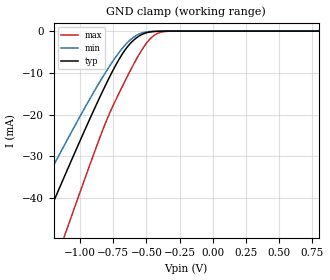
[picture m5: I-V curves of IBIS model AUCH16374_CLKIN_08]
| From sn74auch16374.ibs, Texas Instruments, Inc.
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[Model]   AUCH16374_CLKIN_08
Model_type  Input
Vinl=0
Vinh=0.8
| variable   typ   min   max
C_comp   2.55pF   2.23pF   2.86pF
[Temperature Range]   40   100   -40
| Ambient temperature   25   85   -40
[Voltage range]   0.8   0.8   0.8
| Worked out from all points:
|   GND clamp passes 1 mA (typ) near -0.55 V on its own axis
[GND Clamp]
| AUCH16374_CLKIN_08
|   Voltage   I(typ)   I(min)   I(max)
-3.6V     -222.3mA   -186.1mA   -267.5mA
-1.455V   -59.66mA   -47.61mA   -78.99mA
-1.32V    -49.56mA   -39.31mA   -66.95mA
-1.275V   -46.22mA   -36.57mA   -62.93mA
-1.115V   -34.43mA   -26.99mA   -48.63mA
-1.08V    -31.88mA   -24.93mA   -45.51mA
-825mV    -13.98mA   -10.7mA    -23.23mA
-695mV    -6.114mA   -4.621mA   -14.06mA
-580mV    -1.724mA   -1.092mA   -6.949mA
-450mV    -123.7uA   -58.25uA   -1.212mA
-315mV    -2.431uA   -1.513uA   -21.15uA
800mV     96.17pA    179.1pA    76.88pA
